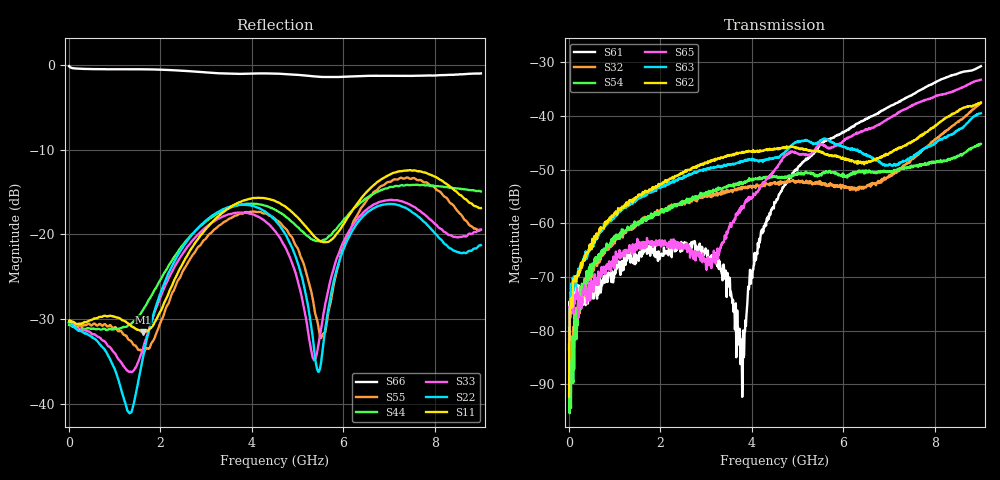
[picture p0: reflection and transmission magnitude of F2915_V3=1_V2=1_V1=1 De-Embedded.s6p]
! Integrated Device Technology
! Corporate Headquarters
! 6024 Silver Creek Valley Road
! San Jose, CA 95138  USA
! Phone:  1-408-284-8200
! Toll Free:  1-800-223-1366
! Webpage:  http://www.idt.com/
! Timing and RF Division
! 515 Groton Road, Suite 102
! Westford, MA 01886-6024
! Device:  F2915
! Description: High Reliability SP5T RF Switch
! Frequency:  0.05 -  8.GHz
! Package:  4x4 mm Thin QFN Plastic Package: 24 pin
! Ports:  6 RF,  5 DC
!  Pin  1  = GND
!  Pin  2  = RF5  =  Port 5
!  Pin  3  = GND
!  Pin  4  = GND
!  Pin  5  = RF4  =  Port 4
!  Pin  6  = GND
!  Pin  7  = GND
!  Pin  8  = RF3  =  Port 3
!  Pin  9  = GND
!  Pin 10  = GND
!  Pin 11  = RF2  =  Port 2
!  Pin 12  = GND
!  Pin 13  = GND
!  Pin 14  = RF1  =  Port 1
!  Pin 15  = GND
!  Pin 16  = Vcc
!  Pin 17  = V1
!  Pin 18  = V2
!  Pin 19  = V3
!  Pin 20  = VSSext
!  Pin 21  = GND
!  Pin 22  = RFC  =  Port 6
!  Pin 23  = GND
!  Pin 24  = GND
! Voltage:  VDD  =  +3.30 Volts
!  VSSEXT =  0.00 Volts
! Current:  IDD  = 297  uA
! State:  All OFF
! V1:  Logic HIGH
! V2:  Logic HIGH
! V3:  Logic HIGH
! Data:  The device was measured on the F291x evaluation board which has
!  individual transmission lines to the RF pins.  Data was collected
!  using a calibrated network analyzer.  The input lines were
!  modeled using Automatic Fixture Removal (AFR) from Keysight.
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# Hz S  dB  R 50
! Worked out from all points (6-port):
!   900 points, 10 MHz to 9 GHz, reference 50 ohm
!   strongest paths, dB at 10 MHz, 2.26 GHz, 4.51 GHz, 6.76 GHz, 9 GHz:
!     S62: -92.3, -51.5, -46.1, -47.8, -37.5
!     S63: -81.7, -52.3, -47.7, -48.2, -39.5
!     S65: -79.3, -63.9, -49.9, -41.6, -33.2
!     S54: -82.5, -56.9, -51.4, -50.4, -45.2
!     S32: -90.1, -56.7, -52.3, -52.1, -37.6
!     S61: -83.5, -64.6, -56.1, -39.4, -30.7
!   lowest |S11| = -31.5 dB at 1.62 GHz (marker M1), VSWR 1.05, Z = 49.5 + j2.6 ohm
!   |S11| at or under -10 dB: start of sweep to end of sweep
